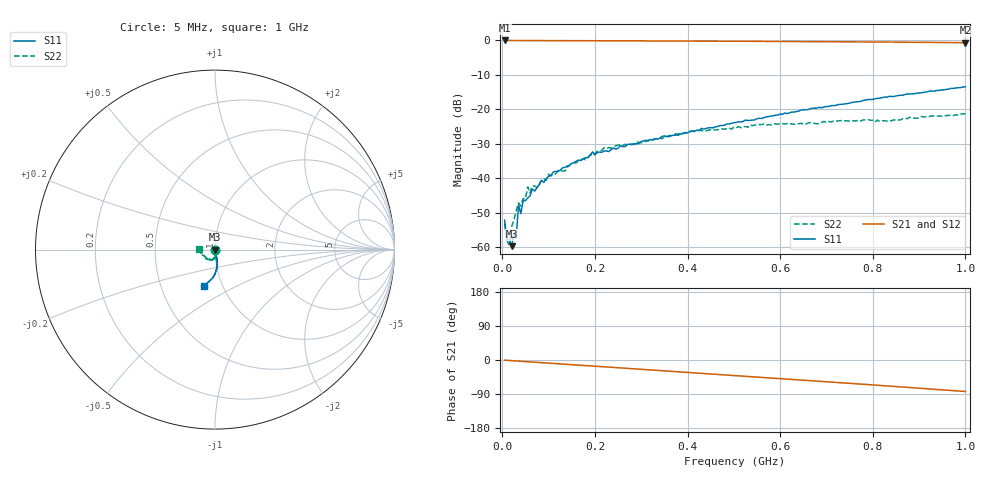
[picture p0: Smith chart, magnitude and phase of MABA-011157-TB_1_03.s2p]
!Agilent Technologies,E5071C,MY46110647,A.11.31
!Date: Thu May 18 15:52:21 2023 DD
!Data & Calibration Information:
!MABA-011157 soldered onto PT-003991 with F connectors, Calibration PCB PT-0003653. Por1 (pin4) Port2 (pin3)
!Freq	S11:SOLT2(ON)	S21:SOLT2(ON)	S12:SOLT2(ON)	S22:SOLT2(ON)
!PortZ  Port1:75+j0  Port2:75+j0
!Above PortZ is port z conversion or system Z0 setting when saving the data.
!When reading, reference impedance value at option line is always used.
# Hz S MA R 75
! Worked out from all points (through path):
!   200 points, 5 MHz to 1 GHz, reference 75 ohm
!   highest |S21| = 0.01 dB at 5 MHz (marker M1); lowest = -0.6 dB at 1 GHz (marker M2)
!   group delay of S21, straight-line fit = 229 ps
!   lowest |S11| = -59.7 dB at 20 MHz (marker M3), VSWR 1.00, Z = 74.9 - j0.0981 ohm
!   |S11| at or under -10 dB: start of sweep to end of sweep
!   |S22| runs from -59.4 to -21.3 dB; largest |S21 - S12| = 0.0056
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5000000  0.002489 -157.3  1.001 -0.5  1.003 -0.4  0.002191 -158.7
1e7  0.00127 -158.6  1 -0.9  1 -0.9  0.001262 160.3
1.5e7  0.001293 -167.5  0.9997 -1.3  0.9997 -1.3  0.001075 -98.5
2e7  0.00104 -141.0  0.9992 -1.8  0.9995 -1.7  0.001997 -100.5
2.5e7  0.00159 -97.8  0.9987 -2.2  0.9991 -2.2  0.002487 -83.5
3e7  0.001361 -101.4  0.9988 -2.6  0.9984 -2.6  0.003351 -71.4
3.5e7  0.004133 -62.2  0.9981 -3.0  0.9988 -3.0  0.004409 -74.2
4e7  0.003082 -64.2  0.998 -3.4  0.9981 -3.4  0.003973 -76.9
4.5e7  0.004807 -74.5  0.9975 -3.8  0.9978 -3.8  0.005082 -70.9
5e7  0.004756 -62.6  0.9975 -4.2  0.9977 -4.2  0.005118 -70.2
5.5e7  0.005217 -63.8  0.997 -4.6  0.9975 -4.6  0.007536 -67.7
6e7  0.00557 -67.9  0.9968 -5.0  0.9974 -5.0  0.006175 -82.6
6.5e7  0.007002 -79.5  0.9968 -5.5  0.9965 -5.4  0.007781 -63.1
7.5e7  0.007309 -64.4  0.9964 -6.3  0.9964 -6.2  0.007354 -74.4
8.5e7  0.009377 -67.5  0.9953 -7.1  0.9961 -7.1  0.009579 -63.6
1.75e8  0.01944 -77.6  0.9925 -14.4  0.9924 -14.3  0.01915 -85.3
2.2e8  0.02502 -80.6  0.9904 -18.0  0.9906 -18.0  0.02789 -84.9
3.4e8  0.03814 -79.2  0.9844 -27.7  0.984 -27.8  0.03914 -90.3
5.05e8  0.06477 -78.1  0.974 -41.2  0.9735 -41.2  0.0541 -103.0
6.7e8  0.1039 -84.2  0.962 -54.8  0.9604 -54.9  0.0635 -119.9
8.35e8  0.1546 -93.3  0.9482 -68.8  0.9438 -68.8  0.06932 -146.2
1e9  0.2133 -107.1  0.9295 -83.1  0.9246 -83.0  0.08649 178.0
